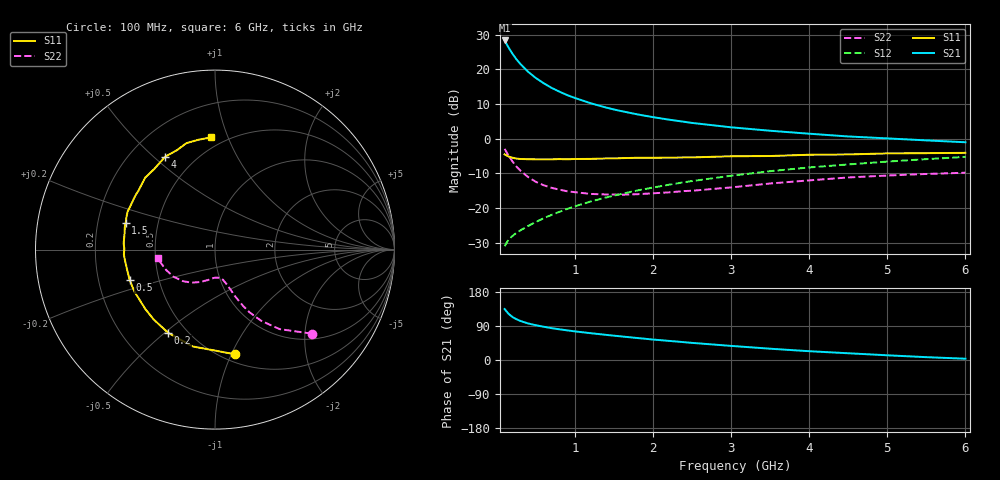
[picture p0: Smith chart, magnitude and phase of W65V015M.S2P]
! SIEMENS Small Signal Semiconductors
! BFR193W
! Si NPN RF Bipolar Junction Transistor in SOT323
! VCE = 5 V  IC = 15 mA
! Common Emitter S-Parameters:  September  1992
# GHz  S  MA  R  50
!  f  S11  S21  S12  S22
! GHz  MAG  ANG  MAG  ANG  MAG  ANG  MAG  ANG
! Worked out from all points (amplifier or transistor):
!   28 points, 100 MHz to 6 GHz, reference 50 ohm
!   highest |S21| = 28.3 dB at 100 MHz (marker M1)
!   |S21| within 3 dB of that: start of sweep to 177.3 MHz
!   unconditionally stable (mu >= 1): 864 MHz to 2.554 GHz
!   at 300 MHz: K = 0.68, MSG = 24.0 dB, |S12| = -26.5 dB
!   at 1.5 GHz: K = 1.04, MAG = 11.2 dB, |S12| = -16.4 dB
!   at 6 GHz: K = 0.90, MSG = 2.1 dB, |S12| = -5.2 dB
!   S11 on the Smith chart (normalised r, x): 100 MHz: 0.57, -1.03; 200 MHz: 0.40, -0.51; 500 MHz: 0.34, -0.15; 1.5 GHz: 0.32, +0.13; 4 GHz: 0.34, +0.54; 6 GHz: 0.42, +0.87
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0.1  0.5937 -79.2  26.13 134.4  0.0282 59.5  0.7136 -41.0
0.15  0.5537 -103.0  20.7 122.0  0.035 54.6  0.571 -50.9
0.2  0.532 -119.3  16.85 113.5  0.0395 52.7  0.4718 -57.1
0.25  0.5182 -131.1  14.05 107.7  0.0438 52.8  0.3979 -61.2
0.3  0.5104 -139.4  12.02 103.2  0.0475 53.7  0.3489 -63.6
0.4  0.5061 -152.4  9.25 96.5  0.0551 56.0  0.2803 -66.9
0.5  0.5048 -160.5  7.508 91.7  0.0629 58.3  0.2391 -68.7
0.6  0.5023 -167.2  6.314 87.7  0.0713 60.3  0.2131 -70.8
0.7  0.5043 -172.1  5.425 84.1  0.0795 61.9  0.1959 -72.1
0.8  0.5085 -176.8  4.783 81.0  0.088 63.1  0.1844 -73.9
0.9  0.5052 179.6  4.263 78.3  0.0972 64.0  0.1746 -75.0
1  0.51 176.1  3.869 75.5  0.1059 64.7  0.1693 -76.6
1.2  0.5117 170.1  3.252 70.8  0.124 65.2  0.1599 -80.8
1.5  0.5195 163.2  2.641 64.2  0.1511 65.4  0.1567 -86.7
1.8  0.5309 156.6  2.244 58.0  0.1792 64.8  0.1584 -92.7
2.2  0.5336 147.9  1.886 50.5  0.2166 63.3  0.1682 -99.9
3  0.5585 134.2  1.461 37.2  0.2921 58.6  0.1986 -114.6
3.5  0.5629 126.7  1.303 29.8  0.3404 54.8  0.226 -125.4
4  0.5873 118.2  1.181 23.2  0.3849 50.7  0.2507 -135.5
4.5  0.5932 110.9  1.078 17.8  0.4256 46.6  0.2761 -146.8
5.5  0.6191 98.5  0.946 7.5  0.5076 38.2  0.3101 -165.9
6  0.6255 91.9  0.889 3.4  0.547 33.6  0.3233 -172.1
